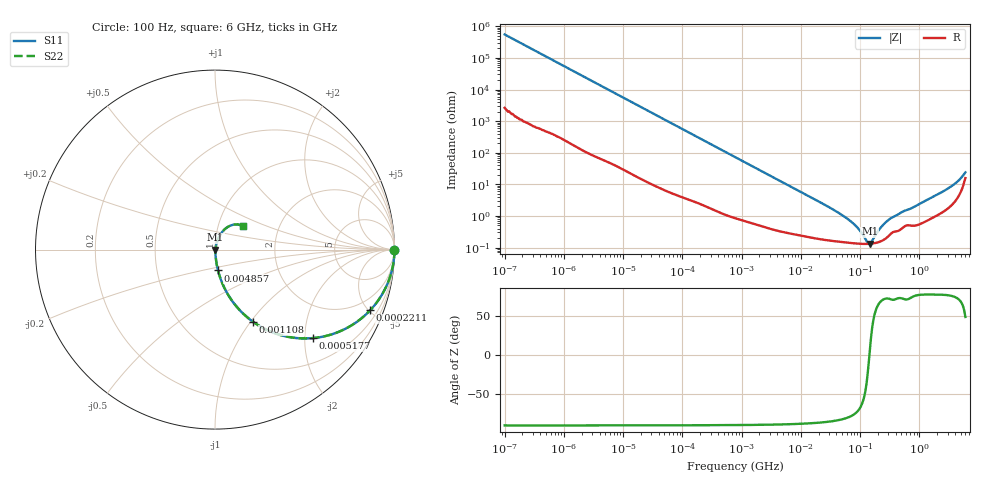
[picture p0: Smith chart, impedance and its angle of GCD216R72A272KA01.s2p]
!Murata Part Number: GCD216R72A272KA01
!These Parameters are Measured in Series Mode Connection
!Data Generated on Jan 08, 2026
!  o--ll--o
!Port1  Port2
!  o------o
!Operation Temp=25[degC], DC Bias Voltage=0[V]
!Freq. Start=100[Hz] Stop=6[GHz] 401[Steps]
# Hz S RI R 50
!Freq.(Hz) S11(Real) S11(Imag) S21(Real) S21(Imag) S12(Real) S12(Imag) S22(Real) S22(Imag)
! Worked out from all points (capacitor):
!   401 points, 100 Hz to 6 GHz, reference 50 ohm
!   read as one part in series: C = 2.88 nF near 109 Hz
!   lowest |Z| = 133 mohm at 145.9 MHz (marker M1)
!   series resonance near 143.8 MHz, so ESL is about 420 pH
!   S11 on the Smith chart (normalised r, x): 100 Hz: open; 221.1 kHz: 1.04, -5.10; 517.7 kHz: 1.02, -2.19; 1.108 MHz: 1.01, -1.03; 4.857 MHz: 1.01, -0.24; 6 GHz: 1.32, +0.36
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100  1 -0.000181  9e-07 0.000181  9e-07 0.000181  1 -0.000181
2008  1 -0.00362  2.91e-05 0.00362  2.91e-05 0.00362  1 -0.00362
40335  0.9944 -0.0716  0.00555 0.0716  0.00555 0.0716  0.9944 -0.0716
112960  0.9599 -0.1925  0.0401 0.1925  0.0401 0.1925  0.9599 -0.1925
221108  0.8648 -0.3377  0.1352 0.3377  0.1352 0.3377  0.8648 -0.3377
330837  0.7431 -0.4324  0.2569 0.4324  0.2569 0.4324  0.7431 -0.4324
517687  0.5447 -0.493  0.4553 0.493  0.4553 0.493  0.5447 -0.493
774597  0.3512 -0.4716  0.6488 0.4716  0.6488 0.4716  0.3512 -0.4716
1108252  0.2118 -0.4019  0.7882 0.4019  0.7882 0.4019  0.2118 -0.4019
2074311  0.0745 -0.2539  0.9255 0.2539  0.9255 0.2539  0.0745 -0.2539
4856642  0.0168 -0.1161  0.9832 0.1161  0.9832 0.1161  0.0168 -0.1161
1.555665e7  0.0034 -0.0369  0.9966 0.0369  0.9966 0.0369  0.0034 -0.0369
6.518806e7  0.00147 -0.00732  0.9985 0.00732  0.9985 0.00732  0.00147 -0.00732
9.326766e7  0.00134 -0.00378  0.9987 0.00378  0.9987 0.00378  0.00134 -0.00378
1.334425e8  0.00131 -0.00064  0.9987 0.00064  0.9987 0.00064  0.00131 -0.00064
1.459435e8  0.00132 0.000129  0.9987 -0.000129  0.9987 -0.000129  0.00132 0.000129
1.596157e8  0.00134 0.000904  0.9987 -0.000904  0.9987 -0.000904  0.00134 0.000904
2.283698e8  0.00162 0.0042  0.9984 -0.0042  0.9984 -0.0042  0.00162 0.0042
3.124326e8  0.0025 0.00744  0.9975 -0.00744  0.9975 -0.00744  0.0025 0.00744
2.802721e9  0.0192 0.0631  0.9808 -0.0631  0.9808 -0.0631  0.0192 0.0631
4.586474e9  0.0534 0.1128  0.9466 -0.1128  0.9466 -0.1128  0.0534 0.1128
6e9  0.1566 0.1308  0.8434 -0.1308  0.8434 -0.1308  0.1566 0.1308
